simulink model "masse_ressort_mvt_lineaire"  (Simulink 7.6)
settings: Solver=ode15s  StartTime=0.0  StopTime=1.5  RelTol=1e-3
InitFcn:
  | B=30;
  | k=1000;
  | m=10;
StopFcn:
  | % lecture du fichier binaire
  | load masse_ressort1.mat
  | close all
  | % trace de la tension et du courant d’induit
  | plotyy(x(1,:),x(2,:), x(1,:),x(3,:))
  | title('Position et vitesse linéaire')
  | grid
  | %axis([0 1.5 -12 12])
libraries: fl_lib x6, nesl_utility x3

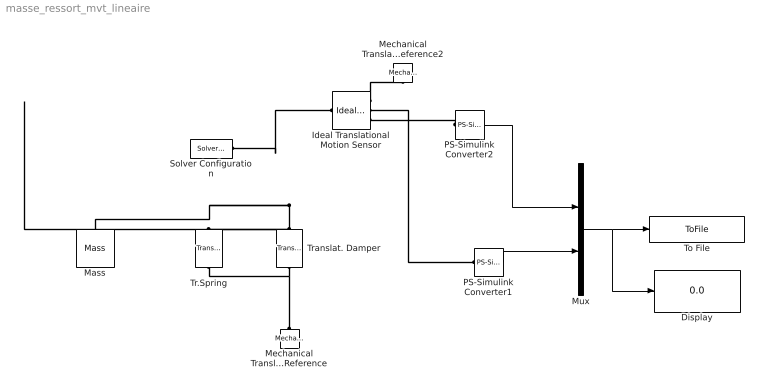
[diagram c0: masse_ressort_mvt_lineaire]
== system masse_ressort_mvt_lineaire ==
  Display : Display
  Ideal Translational Motion Sensor : fl_lib/Mechanical/Mechanical Sensors/Ideal Translational Motion Sensor  DialogController=NetworkEngine.DynNeDlgSource  SystemSampleTime=-1  offset=0 m  v_Log=off  f_Log=off  x_Log=off  LocalVarNames=|v|f|x  LocalVarDescs=|v|f|x  LocalVarLogging=[0 0 0]
  Mass : fl_lib/Mechanical/Translational Elements/Mass  DialogController=NetworkEngine.DynNeDlgSource  SystemSampleTime=-1  mass=m kg  initial_velocity=10 m/s  f_Log=off  LocalVarNames=|f  LocalVarDescs=|f  LocalVarLogging=0
  Mechanical Translational Reference : fl_lib/Mechanical/Translational Elements/Mechanical Translational Reference  DialogController=NetworkEngine.DynNeDlgSource  SystemSampleTime=-1  f_Log=off  LocalVarNames=|f  LocalVarDescs=|f  LocalVarLogging=0
  Mechanical Translational Reference2 : fl_lib/Mechanical/Translational Elements/Mechanical Translational Reference  DialogController=NetworkEngine.DynNeDlgSource  SystemSampleTime=-1  f_Log=off  LocalVarNames=|f  LocalVarDescs=|f  LocalVarLogging=0
  Mux : Mux  Inputs=2
  PS-Simulink Converter1 : nesl_utility/PS-Simulink Converter  DialogController=NetworkEngine.DynNeUtilDlgSource  SystemSampleTime=-1  PhysicalDomain=network_engine_domain  LeftPortType=input  RightPortType=output  SubClassName=ps_output  Unit=1  AffineConversion=off
  PS-Simulink Converter2 : nesl_utility/PS-Simulink Converter  DialogController=NetworkEngine.DynNeUtilDlgSource  SystemSampleTime=-1  PhysicalDomain=network_engine_domain  LeftPortType=input  RightPortType=output  SubClassName=ps_output  Unit=1  AffineConversion=off
  Solver Configuration : nesl_utility/Solver Configuration  DialogController=NetworkEngine.DynNeUtilDlgSource  SystemSampleTime=-1  PhysicalDomain=network_engine_domain  LeftPortType=input  RightPortType=generic  SubClassName=solver  Accelerate=off  Profile=off  ResidualTolerance=1e-9  MaxNonlinIter=12  MaxModeIter=2  DoFixedCost=off  UseLocalSampling=off  DoDC=off  LinearAlgebra=Sparse  LocalSolverSampleTime=.001  LocalSolverChoice=NE_BACKWARD_EULER_ADVANCER  UseLocalSolver=off
  To File : ToFile  Filename=masse_ressort1.mat  MatrixName=x
  Tr.Spring : fl_lib/Mechanical/Translational Elements/Translational Spring  DialogController=NetworkEngine.DynNeDlgSource  SystemSampleTime=-1  spr_rate=k N/m  init_def=0 m  f_Log=off  v_Log=off  x_Log=off  LocalVarNames=|f|v|x  LocalVarDescs=|f|v|x  LocalVarLogging=[0 0 0]
  Translat. Damper : fl_lib/Mechanical/Translational Elements/Translational Damper  DialogController=NetworkEngine.DynNeDlgSource  SystemSampleTime=-1  D=B N/(m/s)  f_Log=off  v_Log=off  LocalVarNames=|f|v  LocalVarDescs=|f|v  LocalVarLogging=[0 0]
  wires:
  PS-Simulink Converter2/1 -> Mux/1
  Mux/1 -> To File/1, Display/1
  PS-Simulink Converter1/1 -> Mux/2
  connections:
  PS-Simulink Converter2/LConn1 -- Ideal Translational Motion Sensor/RConn3
  Ideal Translational Motion Sensor/RConn1 -- Mechanical Translational Reference2/LConn1
  Solver Configuration/RConn1 -- Mass/LConn1 -- Tr.Spring/LConn1 -- Translat. Damper/LConn1 -- Ideal Translational Motion Sensor/LConn1
  Tr.Spring/RConn1 -- Translat. Damper/RConn1 -- Mechanical Translational Reference/LConn1
  Ideal Translational Motion Sensor/RConn2 -- PS-Simulink Converter1/LConn1
